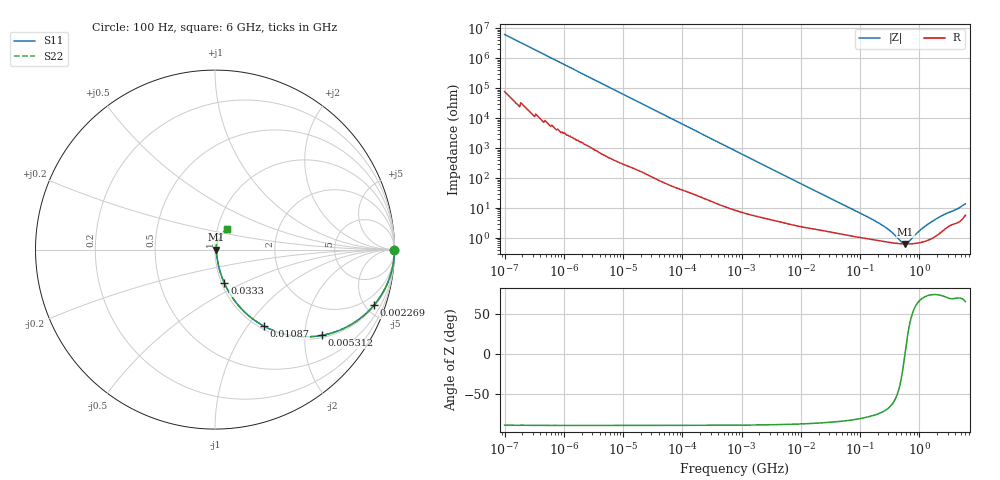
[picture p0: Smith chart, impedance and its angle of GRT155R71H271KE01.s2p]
!Murata Part Number: GRT155R71H271KE01
!These Parameters are Measured in Series Mode Connection
!Data Generated on Jun 19, 2026
!  o--ll--o
!Port1  Port2
!  o------o
!Operation Temp=25[degC], DC Bias Voltage=0[V]
!Freq. Start=100[Hz] Stop=6[GHz] 401[Steps]
# Hz S RI R 50
!Freq.(Hz) S11(Real) S11(Imag) S21(Real) S21(Imag) S12(Real) S12(Imag) S22(Real) S22(Imag)
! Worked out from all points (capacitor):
!   401 points, 100 Hz to 6 GHz, reference 50 ohm
!   read as one part in series: C = 256 pF near 109 Hz
!   lowest |Z| = 641 mohm at 584.8 MHz (marker M1)
!   series resonance near 573.6 MHz, so ESL is about 300 pH
!   S11 on the Smith chart (normalised r, x): 100 Hz: open; 2.269 MHz: 1.09, -5.67; 5.312 MHz: 1.06, -2.44; 10.87 MHz: 1.05, -1.20; 33.3 MHz: 1.03, -0.40; 6 GHz: 1.12, +0.25
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100  1 -1.61e-05  2e-07 1.61e-05  2e-07 1.61e-05  1 -1.61e-05
600  1 -9.61e-05  5e-07 9.61e-05  5e-07 9.61e-05  1 -9.61e-05
2008  1 -0.000321  1.7e-06 0.000321  1.7e-06 0.000321  1 -0.000321
40335  0.9999 -0.00639  7.5e-05 0.00639  7.5e-05 0.00639  0.9999 -0.00639
241822  0.9983 -0.038  0.00174 0.038  0.00174 0.038  0.9983 -0.038
774597  0.9843 -0.1192  0.0157 0.1192  0.0157 0.1192  0.9843 -0.1192
2268635  0.8852 -0.3105  0.1148 0.3105  0.1148 0.3105  0.8852 -0.3105
3394479  0.7784 -0.405  0.2216 0.405  0.2216 0.405  0.7784 -0.405
5311619  0.5959 -0.4778  0.4041 0.4778  0.4041 0.4778  0.5959 -0.4778
7599586  0.4256 -0.479  0.5744 0.479  0.5744 0.479  0.4256 -0.479
1.087309e7  0.2735 -0.4268  0.7265 0.4268  0.7265 0.4268  0.2735 -0.4268
1.555665e7  0.1634 -0.3463  0.8366 0.3463  0.8366 0.3463  0.1634 -0.3463
3.330331e7  0.0523 -0.1872  0.9477 0.1872  0.9477 0.1872  0.0523 -0.1872
1.596157e8  0.0106 -0.0406  0.9894 0.0406  0.9894 0.0406  0.0106 -0.0406
3.124326e8  0.0074 -0.0166  0.9926 0.0166  0.9926 0.0166  0.0074 -0.0166
5.112761e8  0.00641 -0.00304  0.9936 0.00304  0.9936 0.00304  0.00641 -0.00304
5.847788e8  0.00635 0.000518  0.9937 -0.000518  0.9937 -0.000518  0.00635 0.000518
6.688484e8  0.00637 0.00412  0.9936 -0.00412  0.9936 -0.00412  0.00637 0.00412
1.094528e9  0.00752 0.0186  0.9925 -0.0186  0.9925 -0.0186  0.00752 0.0186
1.637704e9  0.0108 0.0337  0.9892 -0.0337  0.9892 -0.0337  0.0108 0.0337
2.450438e9  0.0194 0.0526  0.9806 -0.0526  0.9806 -0.0526  0.0194 0.0526
6e9  0.0679 0.112  0.9321 -0.112  0.9321 -0.112  0.0679 0.112
